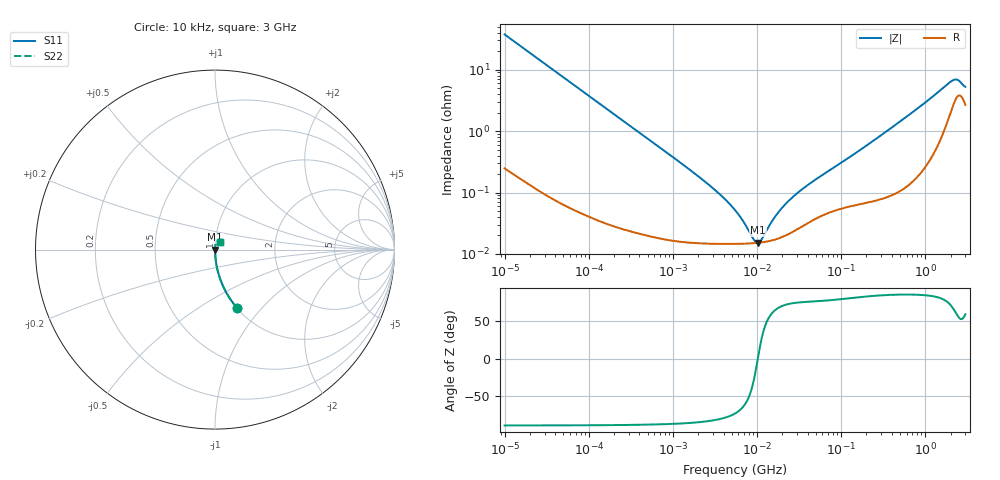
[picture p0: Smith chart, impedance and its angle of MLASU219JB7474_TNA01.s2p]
! MLASU219JB7474_TNA01  S-PARAMETER MODEL  ( Standard Model )
! Model Generated by TAIYO YUDEN Corporation (http://www.ty-top.com)
! Version 1.0
! TAIYO YUDEN Control No. 220601
! Copyright(c) 2011 TAIYO YUDEN CO.,LTD. All Rights Reserved.
! Product Description (link to TY-COMPAS)
! https://ds.yuden.co.jp/TYCOMPAS/or/detail?pn=MLASU219JB7474KTNA01&u=M
! Products Name : Multilayer Ceramic Capacitors
! Characteristics :
!  Capacitance : 0.47 [uF] , Rated Voltage : 50 [V] , TCC : X7R
!  Case Size : 2.0 x 1.25 / 0.079 x 0.049 [mm/inch] , Thickness : 0.85 / 0.033 [mm/inch]
!  (Conditions: Temperature = 25 [degC] , DC Bias Voltage = 0 [V])
! External Node Assignments :
!  1  o---| |---o  2
! GND o---------o GND
! Frequency Range : 10kHz  -  3GHz  [ 401 STEP ]
# MHZ S RI R 50
! Freq[MHz].  S11 Real  S11 Imag  S21 Real  S21 Imag  S12 Real  S12 Imag  S22 Real  S22 Imag
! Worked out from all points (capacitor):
!   401 points, 10 kHz to 3 GHz, reference 50 ohm
!   read as one part in series: C = 426 nF near 10.65 kHz
!   lowest |Z| = 15.2 mohm at 10.29 MHz (marker M1)
!   series resonance near 10.23 MHz, so ESL is about 570 pH
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0.01  0.1236 -0.3259  0.8764 0.3259  0.8764 0.3259  0.1236 -0.3259
0.015549  0.0559 -0.2264  0.9441 0.2264  0.9441 0.2264  0.0559 -0.2264
0.026575  0.0204 -0.1378  0.9796 0.1378  0.9796 0.1378  0.0204 -0.1378
0.082683  0.00251 -0.0453  0.9975 0.0453  0.9975 0.0453  0.00251 -0.0453
0.683653  0.00021 -0.00553  0.9998 0.00553  0.9998 0.00553  0.00021 -0.00553
2.737278  0.000149 -0.00129  0.9999 0.00129  0.9999 0.00129  0.000149 -0.00129
4.124064  0.000146 -0.000776  0.9999 0.000776  0.9999 0.000776  0.000146 -0.000776
5.477226  0.000146 -0.000498  0.9999 0.000498  0.9999 0.000498  0.000146 -0.000498
6.829836  0.000147 -0.000311  0.9999 0.000311  0.9999 0.000311  0.000147 -0.000311
9.070798  0.00015 -9.03e-05  0.9999 9.03e-05  0.9999 9.03e-05  0.00015 -9.03e-05
9.6612  0.000151 -4.29e-05  0.9998 4.29e-05  0.9998 4.29e-05  0.000151 -4.29e-05
10.29003  0.000152 4.41e-06  0.9998 -4.41e-06  0.9998 -4.41e-06  0.000152 4.41e-06
11.31085  0.000154 7.55e-05  0.9998 -7.55e-05  0.9998 -7.55e-05  0.000154 7.55e-05
15.50326  0.000168 0.00032  0.9998 -0.00032  0.9998 -0.00032  0.000168 0.00032
20.5901  0.000193 0.000563  0.9998 -0.000563  0.9998 -0.000563  0.000193 0.000563
29.12589  0.000246 0.000907  0.9998 -0.000907  0.9998 -0.000907  0.000246 0.000907
45.28751  0.000351 0.00145  0.9996 -0.00145  0.9996 -0.00145  0.000351 0.00145
150.0738  0.000643 0.00437  0.9994 -0.00437  0.9994 -0.00437  0.000643 0.00437
374.4521  0.00098 0.0106  0.999 -0.0106  0.999 -0.0106  0.00098 0.0106
2054.98  0.0252 0.0584  0.9748 -0.0584  0.9748 -0.0584  0.0252 0.0584
2405.867  0.038 0.0538  0.962 -0.0538  0.962 -0.0538  0.038 0.0538
3000  0.0279 0.0427  0.9721 -0.0427  0.9721 -0.0427  0.0279 0.0427
